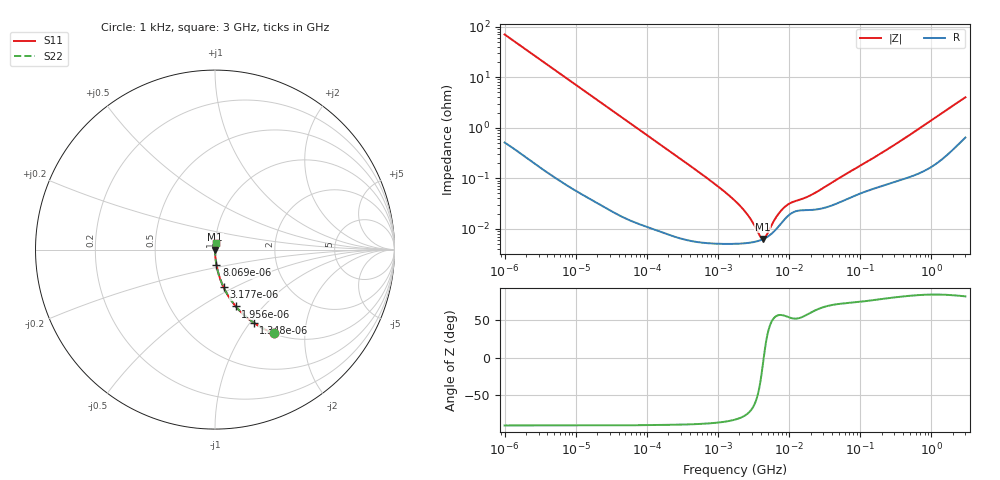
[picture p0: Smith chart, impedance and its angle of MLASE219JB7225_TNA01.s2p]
! MLASE219JB7225_TNA01  S-PARAMETER MODEL  ( Standard Model )
! Model Generated by TAIYO YUDEN Corporation (http://www.ty-top.com)
! Version 1.0
! TAIYO YUDEN Control No. 220601
! Copyright(c) 2009 TAIYO YUDEN CO.,LTD. All Rights Reserved.
! Product Description (link to TY-COMPAS)
! https://ds.yuden.co.jp/TYCOMPAS/or/detail?pn=MLASE219JB7225KTNA01&u=M
! Products Name : Multilayer Ceramic Capacitors
! Characteristics :
!  Capacitance : 2.2 [uF] , Rated Voltage : 16 [V] , TCC : X7R
!  Case Size : 2.0 x 1.25 / 0.079 x 0.049 [mm/inch] , Thickness : 0.85 / 0.033 [mm/inch]
!  (Conditions: Temperature = 25 [degC] , DC Bias Voltage = 0 [V])
! External Node Assignments :
!  1  o---| |---o  2
! GND o---------o GND
! Frequency Range : 1kHz  -  3GHz  [ 401 STEP ]
# MHZ S RI R 50
! Freq[MHz].  S11 Real  S11 Imag  S21 Real  S21 Imag  S12 Real  S12 Imag  S22 Real  S22 Imag
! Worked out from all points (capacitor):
!   401 points, 1 kHz to 3 GHz, reference 50 ohm
!   read as one part in series: C = 2.27 uF near 1.077 kHz
!   lowest |Z| = 6.31 mohm at 4.238 MHz (marker M1)
!   series resonance near 4.392 MHz, so ESL is about 580 pH
!   S11 on the Smith chart (normalised r, x): 1 kHz: 1.01, -1.40; 1.348 kHz: 1.01, -1.04; 1.956 kHz: 1.01, -0.72; 3.177 kHz: 1.00, -0.44; 8.069 kHz: 1.00, -0.18; 3 GHz: 1.01, +0.08
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0.001  0.3297 -0.4665  0.6703 0.4665  0.6703 0.4665  0.3297 -0.4665
0.001348  0.2145 -0.4068  0.7855 0.4068  0.7855 0.4068  0.2145 -0.4068
0.001956  0.1159 -0.3164  0.8841 0.3164  0.8841 0.3164  0.1159 -0.3164
0.003177  0.0481 -0.2105  0.9519 0.2105  0.9519 0.2105  0.0481 -0.2105
0.008069  0.00827 -0.0868  0.9917 0.0868  0.9917 0.0868  0.00827 -0.0868
0.01216  0.00385 -0.0579  0.9961 0.0579  0.9961 0.0579  0.00385 -0.0579
0.033275  0.000672 -0.0214  0.9993 0.0214  0.9993 0.0214  0.000672 -0.0214
0.147855  0.000113 -0.00485  0.9999 0.00485  0.9999 0.00485  0.000113 -0.00485
0.791611  5.22e-05 -0.000884  0.9999 0.000884  0.9999 0.000884  5.22e-05 -0.000884
1.732051  5.06e-05 -0.000355  0.9999 0.000355  0.9999 0.000355  5.06e-05 -0.000355
2.422679  5.19e-05 -0.00021  0.9999 0.00021  0.9999 0.00021  5.19e-05 -0.00021
3.388684  5.58e-05 -8.83e-05  0.9999 8.83e-05  0.9999 8.83e-05  5.58e-05 -8.83e-05
3.651041  5.74e-05 -6.27e-05  0.9999 6.27e-05  0.9999 6.27e-05  5.74e-05 -6.27e-05
4.238263  6.19e-05 -1.21e-05  0.9999 1.21e-05  0.9999 1.21e-05  6.19e-05 -1.21e-05
4.919932  6.92e-05 3.88e-05  0.9999 -3.88e-05  0.9999 -3.88e-05  6.92e-05 3.88e-05
5.30084  7.44e-05 6.45e-05  0.9999 -6.45e-05  0.9999 -6.45e-05  7.44e-05 6.45e-05
7.143107  0.000112 0.000167  0.9999 -0.000167  0.9999 -0.000167  0.000112 0.000167
9.273352  0.000172 0.000237  0.9998 -0.000237  0.9998 -0.000237  0.000172 0.000237
11.1738  0.00021 0.000266  0.9998 -0.000266  0.9998 -0.000266  0.00021 0.000266
21.06097  0.000237 0.000416  0.9998 -0.000416  0.9998 -0.000416  0.000237 0.000416
256.0921  0.000797 0.00387  0.9992 -0.00387  0.9992 -0.00387  0.000797 0.00387
3000  0.00787 0.0388  0.9921 -0.0388  0.9921 -0.0388  0.00787 0.0388
